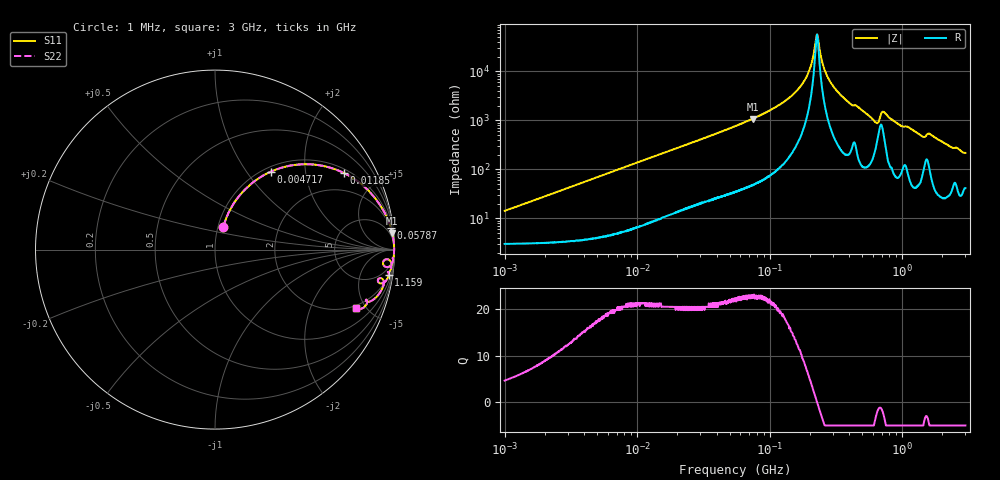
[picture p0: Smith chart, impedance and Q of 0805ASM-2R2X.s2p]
!s-Parameter Generated by FASTRON Sdn. Bhd.
!FASTRON P/N : 0805ASM-2R2X
!Keysight Technologies: E4991B_MY54100416_A.01.15
!Date: Fri Jun 19 14:54:09 2026
!Version  :Rev00  Fri Jun 19 14:54:09 2026
!Data & Calibration Information:
!Freq  S11  S21  S12  S22
!PortZ  Port1:50+j0  Port2:50+j0
!When reading reference impedance value at option line is always used.
! Remarks : This data is being provided solely for informational purposes.
# Hz S dB R 50
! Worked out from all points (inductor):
!   1601 points, 1 MHz to 3 GHz, reference 50 ohm
!   read as one part in series: L = 2.21 uH near 1.041 MHz
!   highest Q = 22.6 at 74.32 MHz (marker M1), where L = 2.3 uH
!   self-resonance near 228 MHz
!   S11 on the Smith chart (normalised r, x): 1 MHz: 1.06, +0.28; 4.717 MHz: 1.08, +1.30; 11.85 MHz: 1.15, +3.25; 57.87 MHz: 2, +16; 1.159 GHz: 2, -13; 3 GHz: 1.83, -4.25
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1000000  -17.30 70.1  -0.34 -7.7  -0.34 -7.7  -17.30 70.1
3804036  -6.86 59.2  -1.30 -26.9  -1.30 -26.9  -6.86 59.2
4717286  -5.47 54.5  -1.77 -32.1  -1.77 -32.1  -5.47 54.5
1.184571e7  -1.57 30.8  -5.79 -56.4  -5.79 -56.4  -1.57 30.8
1.447069e7  -1.15 26.2  -7.08 -61.0  -7.08 -61.0  -1.15 26.2
5.504702e7  -0.12 7.4  -17.80 -80.0  -17.80 -80.0  -0.12 7.4
5.787165e7  -0.11 7.0  -18.20 -80.4  -18.20 -80.4  -0.11 7.0
7.432345e7  -0.07 5.3  -20.70 -82.2  -20.70 -82.2  -0.07 5.3
1.527801e8  -0.02 1.6  -31.00 -84.3  -31.00 -84.3  -0.02 1.6
1.847772e8  -0.02 0.8  -36.70 -82.0  -36.70 -82.0  -0.02 0.8
2.083556e8  -0.02 0.4  -43.80 -73.7  -43.80 -73.7  -0.02 0.4
2.223601e8  -0.02 0.1  -52.20 -44.3  -52.20 -44.3  -0.02 0.1
2.291374e8  -0.02 -0.0  -54.90 11.7  -54.90 11.7  -0.02 -0.0
2.507343e8  -0.02 -0.4  -43.30 74.3  -43.30 74.3  -0.02 -0.4
2.662515e8  -0.02 -0.6  -39.20 79.7  -39.20 79.7  -0.02 -0.6
3.351655e8  -0.02 -1.6  -31.00 83.9  -31.00 83.9  -0.02 -1.6
6.296259e8  -0.31 -5.8  -19.50 67.8  -19.50 67.8  -0.31 -5.8
7.171101e8  -0.24 -3.4  -23.80 62.9  -23.80 62.9  -0.24 -3.4
7.925923e8  -0.12 -4.8  -21.40 78.6  -21.40 78.6  -0.12 -4.8
1.159346e9  -0.19 -8.3  -16.80 77.3  -16.80 77.3  -0.19 -8.3
1.931433e9  -0.43 -14.2  -12.20 71.7  -12.20 71.7  -0.43 -14.2
3e9  -1.43 -22.6  -8.14 56.4  -8.14 56.4  -1.43 -22.6
